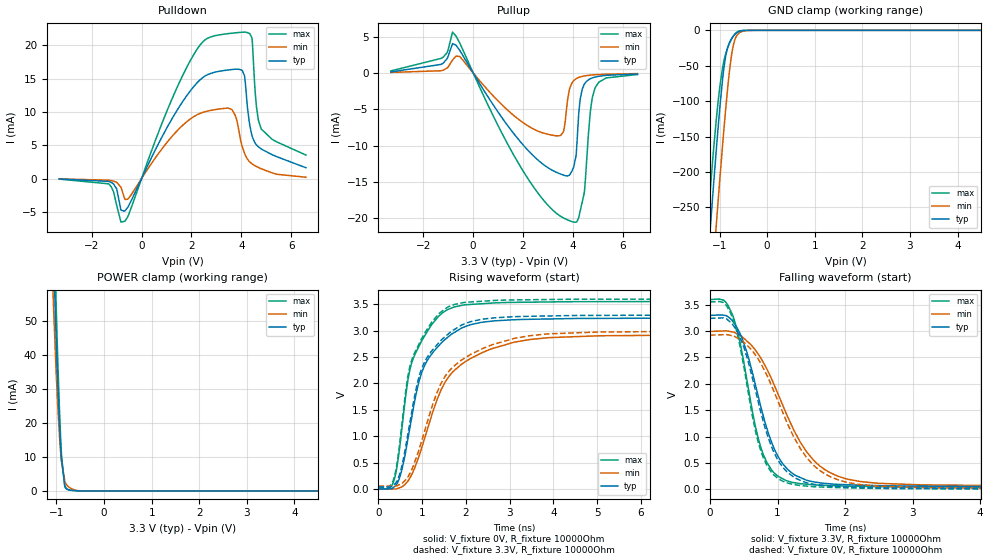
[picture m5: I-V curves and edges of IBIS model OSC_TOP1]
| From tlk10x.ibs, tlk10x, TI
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|   Model
[Model]   OSC_TOP1
Model_type   I/O
Polarity   Non-Inverting
Enable   Active-Low
Vinl = 0.99
Vinh = 2.31
Vmeas = 1.65
Vref = 1.65
Cref = 1pF
Rref = 10000
|   typ   min   max
C_comp   1.479pF   1.451pF  1.549pF
[Voltage Range]   3.3   3   3.6
[Temperature Range]   25   125   -40
[Pullup Reference]   3.3   3   3.6
[Pulldown Reference]   -0   -0   -0
[Power Clamp Reference]   3.3   3   3.6
[GND Clamp Reference]   -0   -0   -0
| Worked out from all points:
|   slope of the pulldown table from 0 to 0.495 V, typ, clamps not added: 128 ohm
|   slope of the pullup table from 0 to 0.495 V, typ, clamps not added: 179 ohm
|   GND clamp passes 1 mA (typ) near -0.56 V on its own axis
|   POWER clamp passes 1 mA (typ) near -0.80 V on its own axis
|   falling waveform, V_fixture 3.3V, R_fixture 10000Ohm: 20-80 % time 446ps typ, 684ps min, 337ps max; typ from 3.3 V to 0.043 V
|   rising waveform, V_fixture 0V, R_fixture 10000Ohm: 20-80 % time 640ps typ, 951ps min, 539ps max; typ from 0.002 V to 3.24 V
|   rising waveform, V_fixture 3.3V, R_fixture 10000Ohm: 20-80 % time 651ps typ, 955ps min, 544ps max; typ from 0.042 V to 3.29 V
|   falling waveform, V_fixture 0V, R_fixture 10000Ohm: 20-80 % time 439ps typ, 669ps min, 333ps max; typ from 3.24 V to 0.002 V
[Pulldown]
|   Voltage   I(typ)   I(min)   I(max)
-3.3V     -71.66uA   -52.19uA   -88.7uA
-1.33V    -430.1uA   -247.6uA   -791.5uA
-825mV    -4.753mA   -1.305mA   -6.55mA
-656.7mV  -4.806mA   -3.141mA   -6.344mA
2.095V    13.81mA    9.285mA    18.62mA
3.472V    16.28mA    10.56mA    21.73mA
3.887V    16.39mA    7.465mA    21.9mA
4.125V    15.44mA    3.824mA    21.96mA
4.422V    6.488mA    2.217mA    21.12mA
4.61V     5.034mA    1.791mA    10.63mA
4.798V    4.423mA    1.465mA    7.426mA
6.59V     1.613mA    192.8uA    3.519mA
[GND Clamp]
|   Voltage   I(typ)   I(min)   I(max)
-3.3V     -2.326A    -2.431A    -2.267A
-1.251V   -331.2mA   -441.1mA   -274.3mA
-1.142V   -233mA     -341.4mA   -181.9mA
-1.063V   -164.8mA   -270.5mA   -122.5mA
-993.3mV  -109.5mA   -210.4mA   -80.02mA
-933.9mV  -68.25mA   -160.9mA   -52.4mA
-864.6mV  -34.17mA   -107mA     -31.64mA
-795.3mV  -17.96mA   -60.32mA   -19.14mA
-735.9mV  -10.75mA   -30.35mA   -10.99mA
-676.5mV  -5.818mA   -13.07mA   -5.093mA
-607.2mV  -2.282mA   -4.919mA   -1.467mA
6.59V     0A         0A         0A
[Pullup]
|   Voltage   I(typ)   I(min)   I(max)
-3.3V     132.3uA    65.1uA     272.7uA
-1.211V   1.312mA    365uA      2.135mA
-825mV    4.033mA    1.762mA    5.619mA
1.67V     -8.528mA   -5.977mA   -11.56mA
3.293V    -13.61mA   -8.645mA   -19.2mA
3.62V     -14.07mA   -8.069mA   -19.96mA
3.858V    -14.08mA   -2.343mA   -20.34mA
4.125V    -11.43mA   -811.4uA   -20.55mA
4.372V    -2.259mA   -480.1uA   -17.81mA
4.709V    -782.5uA   -303.1uA   -5.045mA
4.887V    -569.9uA   -252.6uA   -2.08mA
6.59V     -151.7uA   -94.91uA   -223.2uA
[POWER Clamp]
|   Voltage   I(typ)   I(min)   I(max)
-3.3V     1.531A     1.447A     1.6A
-1.082V   80.47mA    62.78mA    96.82mA
-1.063V   70.57mA    55.01mA    85.38mA
-1.053V   65.79mA    51.28mA    79.78mA
-1.013V   47.9mA     37.42mA    58.41mA
-973.5mV  32.26mA    25.42mA    39.24mA
-933.9mV  19.21mA    15.67mA    23.04mA
-894.3mV  9.395mA    8.676mA    10.66mA
-825mV    1.642mA    2.938mA    1.309mA
-775.5mV  542.6uA    1.64mA     481.5uA
-409.2mV  1.688uA    6.38uA     834.2nA
6.59V     0A         0A         0A
[Ramp]
R_load = 10000
|   typ   min   max
dV/dt_r   1.94197/6.39858e-10   1.75009/9.48741e-10   2.12867/5.37328e-10
dV/dt_f   1.95188/4.45307e-10   1.76247/6.82695e-10   2.1365/3.36756e-10
[Falling Waveform]
V_fixture = 3.3V
V_fixture_min = 3V
V_fixture_max = 3.6V
R_fixture = 10000Ohm
C_fixture = 0F
|   Time   V(typ)   V(min)   V(max)
0s        3.296V     2.992V     3.596V
237.9ps   3.292V     3.002V     3.54V
419.2ps   3.016V     2.932V     2.927V
566.6ps   2.506V     2.786V     1.925V
755.3ps   1.55V      2.48V      782mV
928.5ps   834.7mV    2.042V     339.9mV
1.124ns   415.1mV    1.452V     166.6mV
1.579ns   131.5mV    493mV      79.78mV
2.231ns   78.16mV    145.8mV    55.68mV
8ns       42.52mV    54.25mV    35.29mV
[Rising Waveform]
V_fixture = 0V
V_fixture_min = 0V
V_fixture_max = 0V
R_fixture = 10000Ohm
C_fixture = 0F
|   Time   V(typ)   V(min)   V(max)
0s        1.873mV    3.369mV    1.788mV
366.5ps   42.45mV    -301.7uV   192mV
543.2ps   388.6mV    43.51mV    1.195V
674.5ps   948.7mV    149.6mV    2.07V
793.3ps   1.504V     329.8mV    2.466V
1.08ns    2.378V     1.021V     2.93V
1.571ns   2.863V     2.083V     3.392V
2.354ns   3.155V     2.574V     3.507V
3.461ns   3.213V     2.829V     3.537V
8ns       3.239V     2.92V      3.55V
[Rising Waveform]
V_fixture = 3.3V
V_fixture_min = 3V
V_fixture_max = 3.6V
R_fixture = 10000Ohm
C_fixture = 0F
|   Time   V(typ)   V(min)   V(max)
0s        42.26mV    53.6mV     35.17mV
366.5ps   89.44mV    54.97mV    237.4mV
543.2ps   462.5mV    108mV      1.276V
674.5ps   1.042V     229mV      2.142V
774.3ps   1.518V     392.1mV    2.472V
1.046ns   2.39V      1.068V     2.93V
1.578ns   2.922V     2.195V     3.441V
2.354ns   3.213V     2.648V     3.554V
3.461ns   3.27V      2.902V     3.583V
8ns       3.295V     2.991V     3.596V
[Falling Waveform]
|Gnd
V_fixture = 0V
V_fixture_min = 0V
V_fixture_max = 0V
R_fixture = 10000Ohm
C_fixture = 0F
|   Time   V(typ)   V(min)   V(max)
0s        3.239V     2.921V     3.55V
251.3ps   3.223V     2.93V      3.468V
419.2ps   2.949V     2.857V     2.864V
627.1ps   2.11V      2.621V     1.392V
755.3ps   1.444V     2.375V     714.8mV
928.5ps   750.5mV    1.908V     293.3mV
1.124ns   351mV      1.313V     128.4mV
1.579ns   86.11mV    402.3mV    45.18mV
2.231ns   35.31mV    87.16mV    21.82mV
8ns       2.113mV    3.962mV    1.9mV
